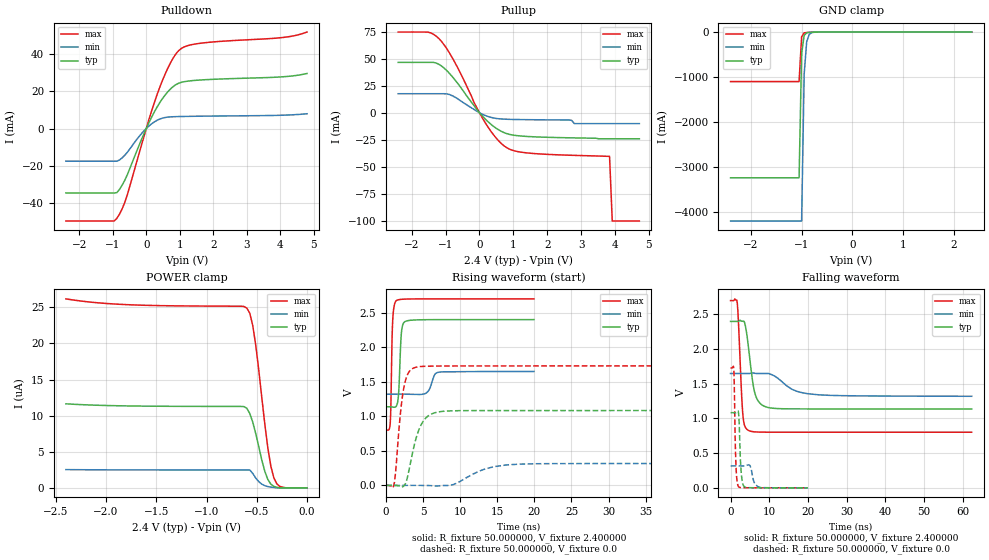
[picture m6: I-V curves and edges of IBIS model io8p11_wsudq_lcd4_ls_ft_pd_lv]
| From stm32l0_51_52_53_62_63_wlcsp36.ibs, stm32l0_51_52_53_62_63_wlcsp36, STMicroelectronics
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|   Model io8p11_wsudq_lcd4_ls_ft_pd_lv
[Model]  io8p11_wsudq_lcd4_ls_ft_pd_lv
Model_type I/O
Polarity   Non-Inverting
Enable   Active-Low
Vinl =   0.720000V
Vinh =   1.680000V
Vmeas =  1.200000V
Cref =   50.000000pF
Rref =   100.000000M
Vref =   0.0V
C_comp   3.178800pF   3.170000pF   3.206700pF
[Temperature Range]   25.000000   0.105000k   -40.000000
[Pullup Reference]   2.400000V   1.650000V   2.700000V
[Pulldown Reference]   0.0V   0.0V   0.0V
[POWER Clamp Reference]   2.400000V   1.650000V   2.700000V
[GND Clamp Reference]   0.0V   0.0V   0.0V
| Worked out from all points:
|   slope of the pulldown table from 0 to 0.36 V, typ, clamps not added: 28.5 ohm
|   slope of the pullup table from 0 to 0.36 V, typ, clamps not added: 32.2 ohm
|   GND clamp passes 1 mA (typ) near -0.64 V on its own axis
|   rising waveform, R_fixture 50.000000, V_fixture 2.400000: 20-80 % time 299ps typ, 648ps min, 215ps max; typ from 1.14 V to 2.4 V
|   rising waveform, R_fixture 50.000000, V_fixture 0.0: 20-80 % time 1.6ns typ, 3.85ns min, 944ps max; typ from 0 V to 1.08 V
|   falling waveform, R_fixture 50.000000, V_fixture 2.400000: 20-80 % time 1.82ns typ, 5.37ns min, 922ps max; typ from 2.4 V to 1.14 V
|   falling waveform, R_fixture 50.000000, V_fixture 0.0: 20-80 % time 495ps typ, 872ps min, 394ps max; typ from 1.08 V to 0 V
[Pulldown]
|Voltage   I(typ)   I(min)   I(max)
-2.4V     -34.71mA   -17.6mA    -49.82mA
-960mV    -34.71mA   -17.6mA    -49.82mA
-880mV    -34.55mA   -17.6mA    -48.46mA
-720mV    -30.52mA   -15.8mA    -43.27mA
-560mV    -24.65mA   -12.68mA   -35.33mA
0V        326fA      0A         10fA
400mV     13.84mA    5.066mA    22.03mA
720mV     21.25mA    6.254mA    35.26mA
1.04V     24.83mA    6.464mA    43.03mA
1.6V      26.11mA    6.627mA    45.88mA
4V        27.76mA    7.125mA    48.88mA
4.8V      29.63mA    7.94mA     51.96mA
[Pullup]
|Voltage   I(typ)   I(min)   I(max)
-2.4V     46.57mA    17.61mA    74.62mA
-1.52V    46.57mA    17.61mA    74.5mA
-1.2V     44.84mA    17.61mA    68.61mA
-720mV    30.25mA    14.38mA    46.12mA
-160mV    6.59mA     3.051mA    9.467mA
160mV     -5.477mA   -2.361mA   -8.695mA
480mV     -14.04mA   -5.167mA   -22.91mA
800mV     -19.2mA    -5.978mA   -32.18mA
1.52V     -22.07mA   -6.4mA     -37.42mA
3.84V     -24mA      -10mA      -40.2mA
3.92V     -24mA      -10mA      -100mA
4.72V     -24mA      -10mA      -100mA
[GND_clamp]
|Voltage   I(typ)   I(min)   I(max)
-2.4V     -3.238A    -4.199A    -1.101A
-1.05V    -3.238A    -4.199A    -1.101A
-1V       -476.5mA   -4.199A    -104.7mA
-950mV    -76.69mA   -936.1mA   -18.75mA
-900mV    -16.87mA   -213.2mA   -9.366mA
-850mV    -6.718mA   -51.14mA   -6.786mA
-800mV    -4.121mA   -13.93mA   -5.004mA
-650mV    -1.082mA   -1.228mA   -1.183mA
2.35V     52.69uA    50.02uA    36.84uA
[POWER_clamp]
|Voltage   I(typ)   I(min)   I(max)
-2.4V     11.64uA    2.527uA    26.18uA
-1.86V    11.37uA    2.49uA     25.43uA
-600mV    11.04uA    2.475uA    24.9uA
-570mV    10.3uA     2.473uA    24.21uA
-540mV    9.097uA    2.001uA    22.48uA
-510mV    7.497uA    1.351uA    19.73uA
-450mV    3.846uA    513.2nA    12.52uA
-390mV    1.155uA    176.1nA    5.528uA
-360mV    508.6nA    103.4nA    2.997uA
-330mV    204.7nA    61.05nA    1.375uA
-270mV    0A         0A         195.3nA
0V        0A         0A         0A
[Ramp]
| variable   typ   min   max
dV/dt_r  0.65004/1.59727n   0.18967/3.84207n   1.03746/0.94021n
dV/dt_f  0.75702/1.81456n   0.19614/5.36002n   1.13800/0.92005n
R_load = 50.000000
[Rising Waveform]
R_fixture= 50.000000
V_fixture= 2.400000
V_fixture_min= 1.650000
V_fixture_max= 2.700000
|time   V(typ)   V(min)   V(max)
0s        1.137V     1.32V      801.8mV
560.6ps   1.137V     1.32V      917.5mV
880.9ps   1.133V     1.32V      2.382V
1.361ns   1.146V     1.32V      2.673V
1.682ns   1.334V     1.32V      2.687V
2.082ns   2.234V     1.32V      2.693V
2.523ns   2.369V     1.32V      2.696V
5.365ns   2.398V     1.334V     2.699V
7.167ns   2.399V     1.639V     2.699V
19.94ns   2.399V     1.649V     2.699V
[Rising Waveform]
R_fixture= 50.000000
V_fixture= 0.0
V_fixture_min= 0.0
V_fixture_max= 0.0
|time   V(typ)   V(min)   V(max)
0s        -2.608uV   4.722uV    224.2uV
1.001ns   110.7uV    1.27uV     -13.11mV
2.002ns   -17.16mV   -4.838uV   1.122V
2.377ns   -8.263mV   10.64uV    1.409V
3.003ns   180.5mV    75.24uV    1.629V
4.004ns   669.4mV    87.61uV    1.71V
5.38ns    978.3mV    -1.501mV   1.724V
8.008ns   1.075V     -1.165mV   1.728V
17.89ns   1.083V     307.2mV    1.729V
62.31ns   1.083V     316.1mV    1.729V
[Falling Waveform]
R_fixture= 50.000000
V_fixture= 2.400000
V_fixture_min= 1.650000
V_fixture_max= 2.700000
|time   V(typ)   V(min)   V(max)
0s        2.399V     1.649V     2.699V
1.752ns   2.398V     1.649V     2.655V
3.128ns   2.402V     1.649V     1.092V
3.754ns   2.355V     1.648V     881.8mV
4.63ns    2.028V     1.649V     828.1mV
5.631ns   1.563V     1.655V     811.3mV
6.381ns   1.347V     1.65V      806.7mV
9.384ns   1.163V     1.648V     802.4mV
19.77ns   1.138V     1.358V     801.8mV
62.31ns   1.137V     1.32V      801.8mV
[Falling Waveform]
R_fixture= 50.000000
V_fixture= 0.0
V_fixture_min= 0.0
V_fixture_max= 0.0
|time   V(typ)   V(min)   V(max)
0s        1.083V     316.1mV    1.729V
840.8ps   1.083V     316.1mV    1.708V
1.201ns   1.083V     316.1mV    699.1mV
1.401ns   1.083V     316.1mV    326.6mV
2.042ns   1.087V     316.1mV    17.57mV
2.723ns   246.4mV    315.9mV    3.843mV
3.483ns   21.91mV    316.4mV    2.12mV
4.925ns   2.457mV    326mV      951.9uV
7.608ns   644.4uV    6.697mV    410.7uV
19.94ns   -2.608uV   4.722uV    224.2uV
